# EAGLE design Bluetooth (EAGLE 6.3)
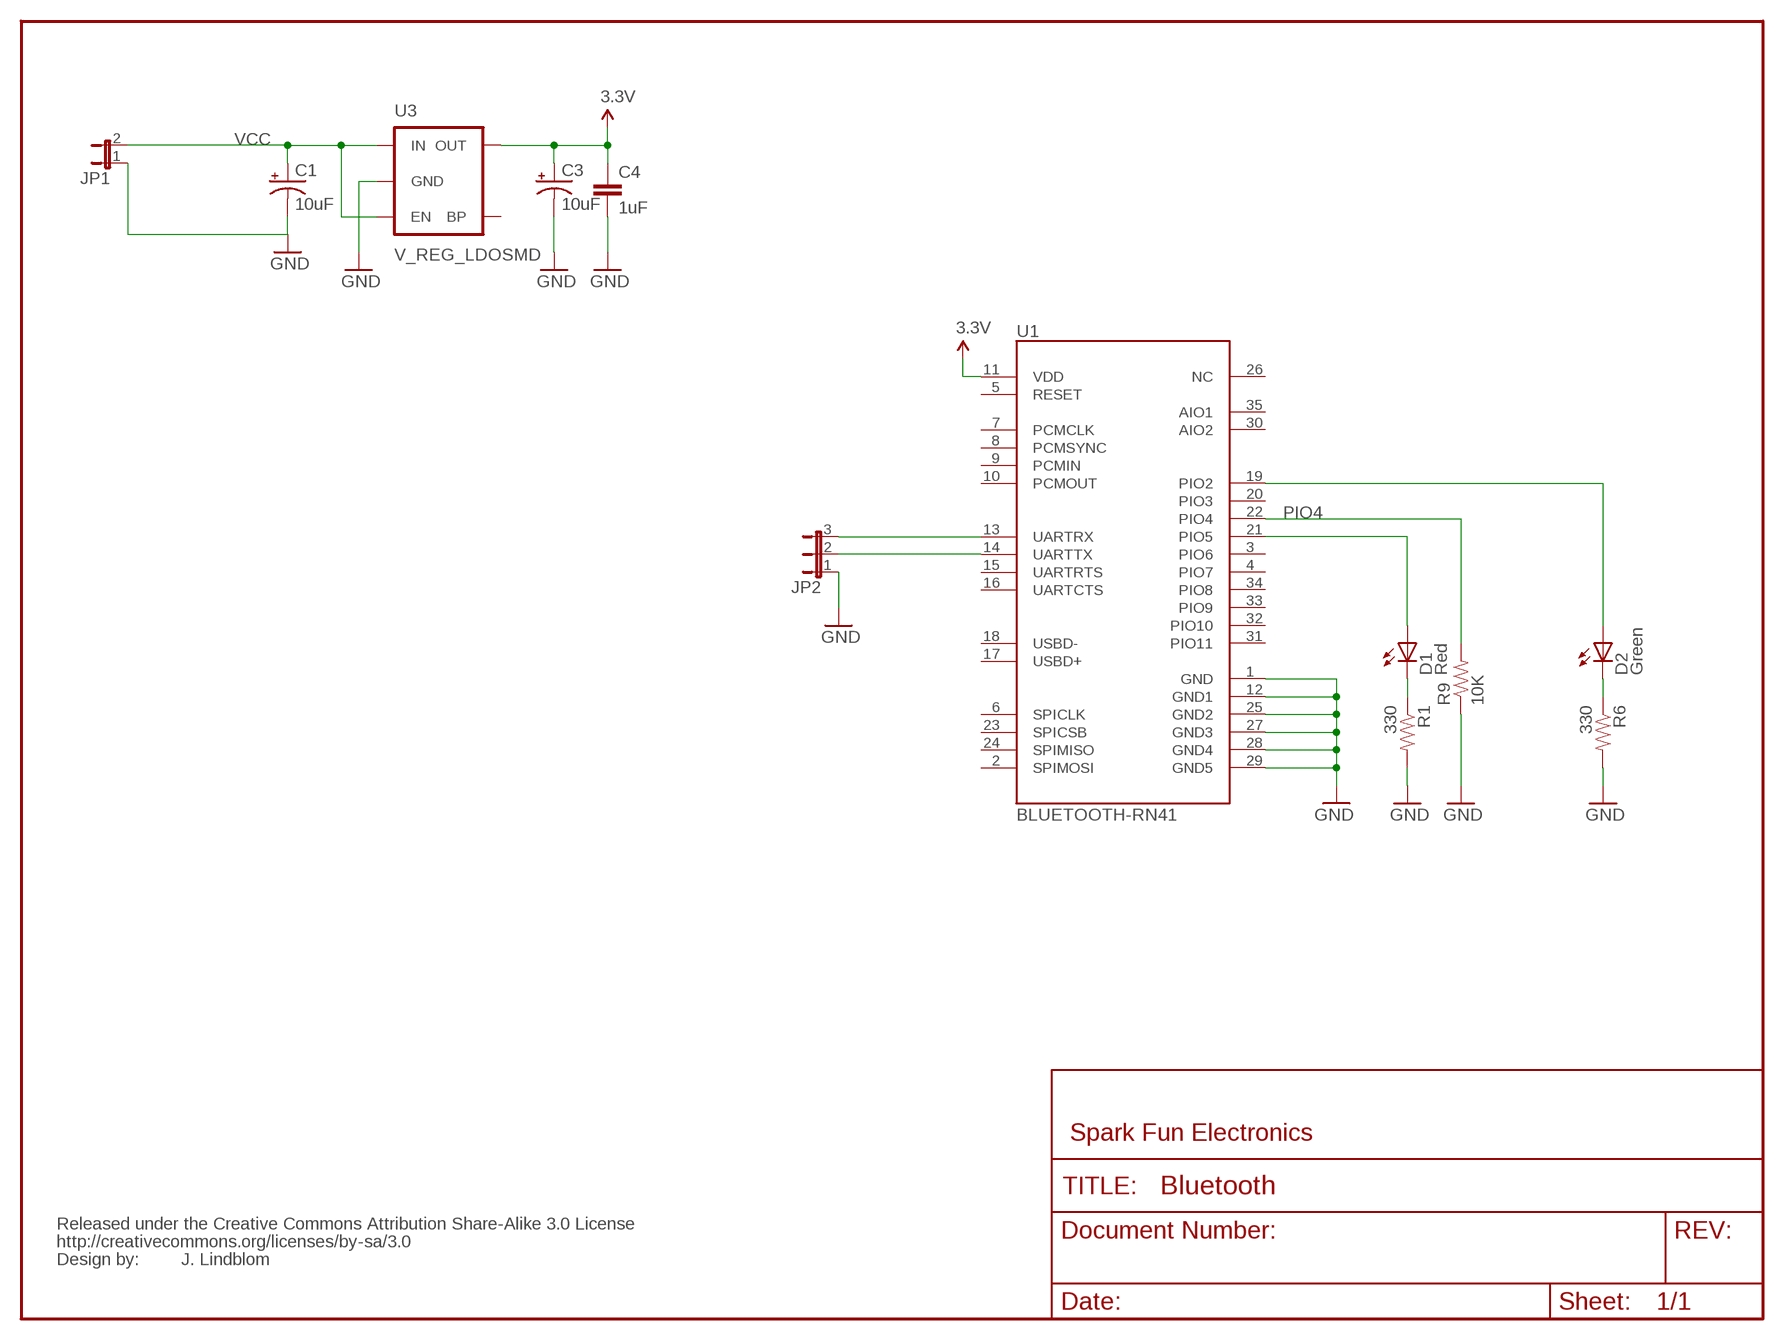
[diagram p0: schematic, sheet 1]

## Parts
C1  10uF  CAP_POL1206  [EIA3216]
C3  10uF  CAP_POL1206  [EIA3216]
C4  1uF  CAP0402-CAP  [0402-CAP]
D1  Red  LED0603  [LED-0603]
D2  Green  LED0603  [LED-0603]
JP1  JP1E  [JP1]
JP2  JP2E  [JP2]
R1  330  RESISTOR0402-RES  [0402-RES]
R6  330  RESISTOR0402-RES  [0402-RES]
R9  10K  RESISTOR0402-RES  [0402-RES]
U1  BLUETOOTH-RN41  BLUETOOTH-RN41"  [RN41]
U3  V_REG_LDOSMD  [SOT23-5]
U$2  CREATIVE_COMMONS  [CREATIVE_COMMONS]

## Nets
3.3V: C3.A(+) C4.1 U1.11(VDD) U3.5(OUT)
D1: D1.C R1.1
D2: D2.C R6.1
GND: C1.C(-) C3.C(-) C4.2 JP1.1 JP2.1 R1.2 R6.2 R9.1 U1.1(GND) U1.12(GND1) U1.25(GND2) U1.27(GND3) U1.28(GND4) U1.29(GND5) U3.2(GND)
N$1: D1.A U1.21(PIO5)
N$2: D2.A U1.19(PIO2)
N$4: JP2.3 U1.13(UARTRX)
N$5: JP2.2 U1.14(UARTTX)
PIO4: R9.2 U1.22(PIO4)
VCC: C1.A(+) JP1.2 U3.1(IN) U3.3(EN)
Unconnected: U1.2(SPIMOSI) U1.3(PIO6) U1.4(PIO7) U1.5(RESET) U1.6(SPICLK) U1.7(PCMCLK) U1.8(PCMSYNC) U1.9(PCMIN) U1.10(PCMOUT) U1.15(UARTRTS) U1.16(UARTCTS) U1.17(USBD+) U1.18(USBD-) U1.20(PIO3) U1.23(SPICSB) U1.24(SPIMISO) U1.26(NC) U1.30(AIO2) U1.31(PIO11) U1.32(PIO10) U1.33(PIO9) U1.34(PIO8) U1.35(AIO1) U3.4(BP)

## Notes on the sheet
- Spark Fun Electronics
- J. Lindblom

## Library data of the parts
C1 C3 = SparkFun:CAP_POL: Capacitor Polarized
C4 = SparkFun:CAP: Capacitor
D1 D2 = SparkFun:LED: LEDs
JP1 = jumper:JP1E: JUMPER
JP2 = jumper:JP2E: JUMPER
R1 R6 R9 = SparkFun:RESISTOR: Resistor
U1 = ScratchPad:BLUETOOTH-RN41
U3 = SparkFun:V_REG_LDO: Voltage Regulator LDO Standard 150mA LDO voltage regulator in SOT-23 layout. Micrel part MIC5205. BP (by-pass) pin is used to lower output noise with 470pF cap.
U$2 = SparkFun:CREATIVE_COMMONS

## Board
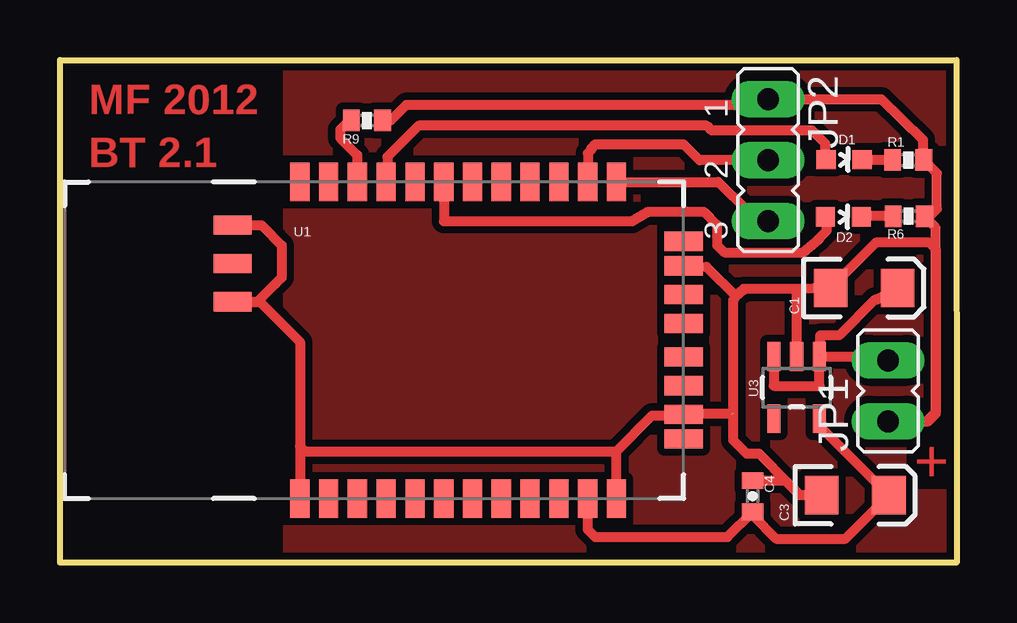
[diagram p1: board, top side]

Size 37.38 x 20.97 mm. Coordinates in mm from the lower left corner, seen from the top.
Outline: 0.01,0 0,20.97 37.37,20.97 37.38,0 0.01,0
Copper layers (1*16): Top 0.035mm / dielectric 1.5mm / Bottom 0.035mm
Design rules "SparkFun": minimum track width 8mil, minimum drill 20mil, track to track 8mil, track to pad 8mil, pad to pad 8mil, via to via 8mil, smd to smd 8mil, copper to edge 9mil, drill to drill 8mil, minimum pad ring 12mil, minimum via ring 10mil, stop-mask expansion 4mil, vias tented up to drill 20mil, thermal gap 10mil

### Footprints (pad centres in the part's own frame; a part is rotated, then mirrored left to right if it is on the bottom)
EIA3216 = smd 1.4 x 1.6: A 1.4,0; C -1.4,0
0402-CAP = smd 0.7 x 0.9: 1 -0.65,0; 2 0.65,0
LED-0603 = smd 0.8 x 0.8: A 0,-0.75; C 0,0.75
JP1 = drill 0.914 long: 1 0,-1.27; 2 0,1.27
JP2 = drill 0.914 long: 1 -2.54,0; 2 0,0; 3 2.54,0
0402-RES = smd 0.7 x 0.9: 1 -0.65,0; 2 0.65,0
RN41 = smd 0.8 x 1.6: 1 -6.6,-6.6; 2 -5.4,-6.6; 3 -4.2,-6.6; 4 -3,-6.6; 5 -1.8,-6.6; 6 -0.6,-6.6; 7 0.6,-6.6; 8 1.8,-6.6; 9 3,-6.6; 10 4.2,-6.6; 11 5.4,-6.6; 12 6.6,-6.6; 13 6.6,6.6; 14 5.4,6.6; 15 4.2,6.6; 16 3,6.6; 17 1.8,6.6; 18 0.6,6.6; 19 -0.6,6.6; 20 -1.8,6.6; 21 -3,6.6; 22 -4.2,6.6; 23 -5.4,6.6; 24 -6.6,6.6 | smd 1.6 x 0.8: 25 -9.4,4.8; 26 -9.4,3.2; 27 -9.4,1.6; 28 9.4,3.1; 29 9.4,-3.1; 30 9.4,-4.122; 31 9.4,-1.9; 32 9.4,-0.7; 33 9.4,0.7; 34 9.4,1.9; 35 9.4,4.122
SOT23-5 = smd 0.55 x 1.2: 1 -0.95,-1.3; 2 0,-1.3; 3 0.95,-1.3; 4 0.95,1.3; 5 -0.95,1.3

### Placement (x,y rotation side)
C1  33.52,11.46 0 top
C3  33.15,2.82 0 top
C4  28.88,2.78 90 top
D1  32.68,16.81 270 top
D2  32.66,14.42 270 top
JP1  34.52,7.17 0 top
JP2  29.52,16.79 270 top
R1  35.36,16.79 0 top
R6  35.38,14.45 0 top
R9  12.79,18.44 180 top
U1  16.6,9.28 0 top
U3  30.71,7.31 180 top
U$2  not placed on the board

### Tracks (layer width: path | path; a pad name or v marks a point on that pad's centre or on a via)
3.3V
  Top 0.406: U1.11 22,1.39 22.31,1.08 27.82,1.08 C4.1 28.88,1.98 29.85,1.01 32.74,1.01 C3.A 31.66,5.71 U3.5
D1
  Top 0.406: R1.1 33.46,16.79 D1.C
D2
  Top 0.406: R6.1 33.44,14.45 D2.C
GND  (1 unrouted)
  Top 0.406: U1.25 8.4,14.08 9.24,13.24 9.24,11.89 8.99,11.64 8.98,11.64 8.22,10.88 U1.27 8.25,10.88 8.34,10.88 10.01,9.21 10.01,4.86 | 10.01,4.86 10.01,2.69 U1.1 | C4.2 28.89,3.42 30.24,3.42 30.84,2.82 C3.C 30.86,2.82 30.33,3.35 29.15,4.55 28.63,4.55 28.07,5.11 28.07,6.14 28,6.18 27.99,6.2 25.5,6.2 U1.29 25.95,6.14 24.68,6.14 23.2,4.65 U1.12 23.2,4.61 23.21,4.63 10.24,4.63 10.01,4.86 | 30.65,11.42 C1.C 34.01,13.35 36.24,13.35 36.53,13.06 36.53,6.31 36.12,5.9 JP1.1 36.2,5.9 36.5,6.2 36.5,13.98 R6.2 36.25,14.45 36.56,14.76 36.56,16.24 R1.2 35.97,16.83 35.97,17.64 34.24,19.33 JP2.1 29.01,19.1 14.44,19.1 13.79,18.44 R9.1 | 30.65,11.42 28.51,11.42 | 28.51,11.42 28.5,11.36 | U1.28 26.95,12.34 28.17,11.12 | 28.07,6.26 28.07,10.94 28.17,11.12 | 28.17,11.12 28.51,11.42 | U3.2 30.71,11.36 30.65,11.42
N$1
  Top 0.406: U1.21 13.65,15.93 13.65,16.93 14.95,18.23 26.96,18.23 27.16,18.03 31.36,18.03 31.9,17.48 D1.A
N$2
  Top 0.406: U1.19 16.01,14.25 23.85,14.25 24.52,14.64 26.84,14.64 27.39,14.09 27.39,13.25 27.7,12.94 30.96,12.94 31.64,13.5 31.64,13.53 31.96,13.85 31.96,14.37 D2.A
N$3
  pour Top (isolate 0.305): 9.41,20.74 37.36,20.74 37.36,-0.06 9.52,-0.06 9.52,20.68
N$4
  Top 0.406: U1.13 27.45,15.88 28.69,14.64 29.1,14.26 JP2.3
N$5
  Top 0.406: JP2.2 26.66,16.79 26.01,17.44 22.31,17.44 22.15,17.28 22.15,17.23 22,17.08 U1.14
PIO4
  Top 0.406: 12.44,15.92 U1.22 12.39,17.01 11.68,17.72 11.68,18.07 12.06,18.44 R9.2
VCC
  Top 0.406: C1.A 34.05,10.98 33.97,10.98 32.48,9.49 31.71,9.49 31.68,9.46 31.68,8.63 U3.1 | U3.3 29.76,7.38 31.66,7.38 U3.1 | U3.1 34.52,8.61 JP1.2

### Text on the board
Top: MF 2012 | BT 2.1 | +

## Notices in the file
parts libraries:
SparkFun: Released under the Creative Commons Attribution Share-Alike 3.0 License
SparkFun: http://creativecommons.org/licenses/by-sa/3.0
